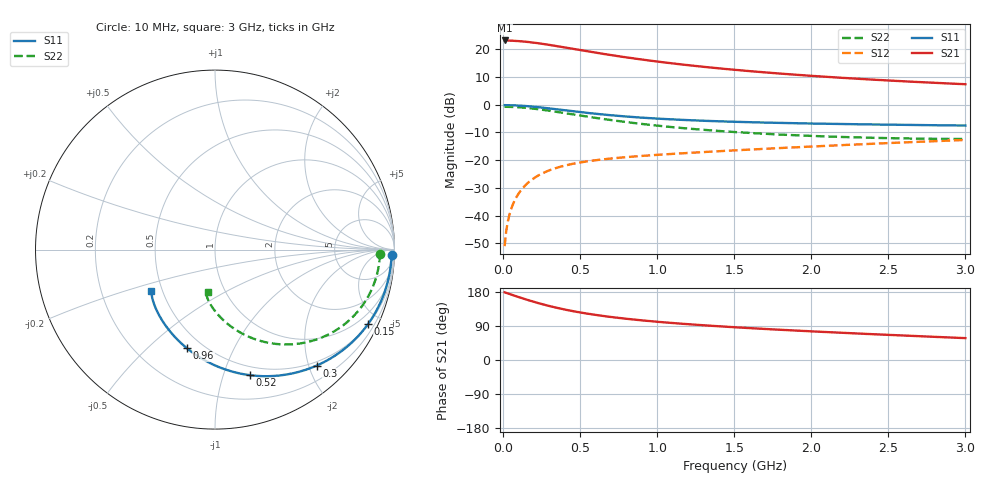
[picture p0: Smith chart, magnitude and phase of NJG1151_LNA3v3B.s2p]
! Created Fri Aug 03 15:19:18 2012
# hz S ma R 50
! 2 Port Network Data LNA section Port1:LNAIN  Port2:LNAOUT  VDD=3.3V,IDD=104mA  LNAIN not connect GND Resistor
! freq  magS11  angS11  magS21  angS21  magS12  angS12  magS22  angS22
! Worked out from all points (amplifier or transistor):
!   300 points, 10 MHz to 3 GHz, reference 50 ohm
!   highest |S21| = 23.2 dB at 10 MHz (marker M1)
!   |S21| within 3 dB of that: start of sweep to 450.7 MHz
!   unconditionally stable (mu >= 1): nowhere
!   at 510 MHz: K = 0.31, MSG = 20.2 dB, |S12| = -20.7 dB
!   at 1.51 GHz: K = 0.69, MSG = 14.5 dB, |S12| = -16.4 dB
!   at 3 GHz: K = 0.88, MSG = 10.1 dB, |S12| = -12.7 dB
!   lowest NFmin = 0.19 dB at 10 MHz
!   S11 on the Smith chart (normalised r, x): 10 MHz: 26, -52; 150 MHz: 0.52, -4.28; 300 MHz: 0.43, -2.13; 520 MHz: 0.42, -1.23; 960 MHz: 0.41, -0.67; 3 GHz: 0.44, -0.24
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1e7  0.9844 -1.8  14.48 178.6  0.002805 61.8  0.9197 -1.4
3e7  0.9831 -5.3  14.44 175.8  0.007584 77.7  0.9183 -4.2
5e7  0.9806 -8.8  14.37 173.0  0.01251 79.9  0.9155 -7.0
1e8  0.9684 -17.5  14.11 166.2  0.02475 78.3  0.902 -13.8
1.5e8  0.9482 -26.0  13.71 159.6  0.03644 74.8  0.8796 -20.5
2.2e8  0.91 -37.2  12.99 151.1  0.05125 69.6  0.8371 -29.2
2.6e8  0.8851 -43.1  12.53 146.7  0.05876 66.8  0.8092 -33.8
3e8  0.8593 -48.8  12.04 142.5  0.06557 64.2  0.7801 -38.1
3.4e8  0.8333 -54.1  11.55 138.6  0.07171 61.9  0.7506 -42.2
3.9e8  0.8015 -60.3  10.95 134.1  0.07855 59.3  0.7142 -46.8
5.1e8  0.732 -73.4  9.612 124.8  0.09187 54.5  0.633 -56.3
5.2e8  0.7268 -74.3  9.508 124.1  0.09282 54.2  0.6268 -57.0
6.2e8  0.6791 -83.4  8.553 117.9  0.1013 51.5  0.5693 -63.4
7.2e8  0.6397 -91.1  7.735 112.5  0.1085 49.6  0.5204 -68.8
8.3e8  0.6044 -98.5  6.974 107.5  0.1153 48.2  0.4753 -73.9
9.6e8  0.5714 -105.9  6.23 102.3  0.1226 47.2  0.4318 -78.9
1.01e9  0.5607 -108.4  5.981 100.6  0.1253 47.0  0.4174 -80.6
1.23e9  0.5237 -117.8  5.079 93.6  0.1366 46.4  0.3661 -87.0
1.51e9  0.4922 -126.8  4.257 86.3  0.1508 46.3  0.3211 -92.8
2.01e9  0.4581 -137.3  3.314 75.4  0.1768 46.3  0.2735 -98.9
2.51e9  0.4369 -143.6  2.733 66.1  0.2042 45.8  0.2495 -100.9
3e9  0.4217 -147.1  2.349 57.7  0.2318 44.5  0.2411 -100.0
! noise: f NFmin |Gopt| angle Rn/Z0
1e+07  0.1871  0.7605  0.5081  0.1578
3.4e+08  0.397  0.5584  17.96  0.1584
6.7e+08  0.701  0.3591  40.1  0.1573
1e+09  1.013  0.25  71.21  0.1551
1.33e+09  1.32  0.2258  106  0.1525
1.67e+09  1.626  0.2507  132.6  0.15
2e+09  1.91  0.2867  149  0.1484
2.33e+09  2.18  0.3198  160.1  0.1485
2.66e+09  2.435  0.3462  168.4  0.1508
3e+09  2.681  0.3658  175.2  0.1565
